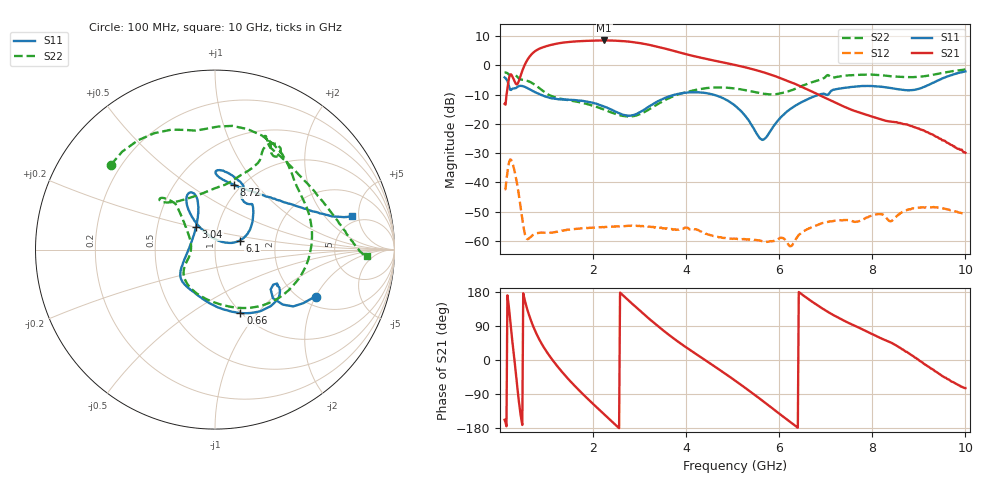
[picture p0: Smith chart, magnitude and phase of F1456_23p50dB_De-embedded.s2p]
! Integrated Device Technology
! Corporate Headquarters
! 6024 Silver Creek Valley Road
! San Jose, CA 95138  USA
! Phone:  1-408-284-8200
! Toll Free:  1-800-223-1366
! Webpage:  http://www.idt.com/
! Timing and RF Division
! 515 Groton Road, Suite 102
! Westford, MA 01886-6024
! Device:  F1456
! Description: 6-bit 0.5 dB Transmit Variable Gain Amplifier
! Frequency:  2100.0 -  2950.00 MHz
! Package:  6x6 mm Thin QFN Plastic Package: 28 pin
! State:  47
! Atten State:  23.5 dB
! Voltage:  +5.00 Volts
! Current:  216.957 mA
! Data:  The device was measured on a the F1455 evaluation board which has
!  individual transmission lines to the RF pins.  Data was collected
!  using a calibrated network analyzer.  The evaluation board was
!  de-embedded using a TRL calibration technique.
!  The reference plane is the edge of the package pin.
!  Pin  1 = CSb
!  Pin  2 = DATA
!  Pin  3 = CLK
!  Pin  4 = RSET
!  Pin  5 = GND
!  Pin  6 = RFIN  = Port 1
!  Pin  7 = GND
!  Pin  8 = NC
!  Pin  9 = NC
!  Pin 10 = NC
!  Pin 11 = NC
!  Pin 12 = NC
!  Pin 13 = NC
!  Pin 14 = /STBY
!  Pin 15 = GND
!  Pin 16 = RFOUT  = Port 2
!  Pin 17 = GND
!  Pin 18 = NC
!  Pin 19 = NC
!  Pin 20 = NC
!  Pin 21 = GND
!  Pin 22 = NC
!  Pin 23 = GND
!  Pin 24 = NC
!  Pin 25 = NC
!  Pin 26 = NC
!  Pin 27 = GND
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# GHz S dB R 50
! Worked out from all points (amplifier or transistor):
!   496 points, 100 MHz to 10 GHz, reference 50 ohm
!   highest |S21| = 8.5 dB at 2.24 GHz (marker M1)
!   |S21| within 3 dB of that: 822.2 MHz to 3.602 GHz (2.78 GHz wide, 126 % of centre)
!   unconditionally stable (mu >= 1): start of sweep to end of sweep
!   at 1.74 GHz: K = 104.57, MAG = 8.8 dB, |S12| = -55.7 dB
!   at 5.06 GHz: K = 365.45, MAG = 1.0 dB, |S12| = -59.2 dB
!   at 10 GHz: K = 590.36, MAG = -20.2 dB, |S12| = -50.8 dB
!   S11 on the Smith chart (normalised r, x): 100 MHz: 2.37, -2.02; 660 MHz: 0.99, -0.82; 3.04 GHz: 0.79, +0.20; 6.1 GHz: 1.31, +0.13; 8.72 GHz: 0.92, +0.77; 10 GHz: 4.18, +4.11
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0.1  -4.14 -24.9  -13.18 -157.8  -42.29 49.7  -2.52 140.8
0.24  -8.43 -31.0  -3.13 79.8  -32.30 -76.4  -3.42 94.5
0.32  -7.91 -29.8  -5.73 -9.6  -36.53 -154.1  -3.25 67.7
0.42  -7.05 -37.0  -4.75 -123.3  -45.72 140.8  -4.66 40.8
0.54  -7.41 -53.7  0.39 154.6  -57.89 130.5  -5.11 16.5
0.66  -8.39 -68.1  3.40 106.2  -58.63 145.0  -5.79 -11.0
0.84  -9.81 -86.8  5.60 55.4  -57.18 116.0  -7.73 -48.8
1.16  -11.41 -113.2  7.17 -5.0  -56.96 78.1  -10.82 -94.5
1.48  -11.76 -130.4  7.95 -51.8  -56.10 55.7  -11.95 -123.2
1.76  -12.13 -140.7  8.25 -87.4  -55.65 40.1  -12.79 -138.9
2.24  -14.09 -156.1  8.46 -143.5  -55.28 19.4  -15.15 -156.0
2.62  -16.77 178.0  8.27 173.3  -54.92 3.5  -17.24 -172.8
3.04  -15.74 130.4  7.46 126.5  -54.88 -15.1  -16.44 157.6
3.4  -12.23 112.4  6.27 88.7  -55.34 -32.0  -13.21 140.1
4.1  -9.21 112.9  3.36 25.2  -56.06 -64.0  -8.80 132.0
5.06  -13.90 125.4  0.06 -55.0  -59.22 -114.4  -7.96 138.0
5.64  -25.50 69.3  -2.30 -107.5  -60.06 -158.8  -9.67 122.2
6.1  -16.73 20.0  -4.86 -151.0  -59.13 164.6  -9.29 89.4
6.7  -10.98 41.3  -8.94 154.4  -55.25 146.6  -5.82 64.9
8.36  -7.69 88.3  -19.15 48.5  -53.08 67.3  -3.72 62.4
8.72  -8.52 73.6  -20.17 21.8  -49.60 69.6  -4.02 50.2
10  -2.09 13.8  -29.86 -74.0  -50.82 -23.7  -1.46 -2.6
